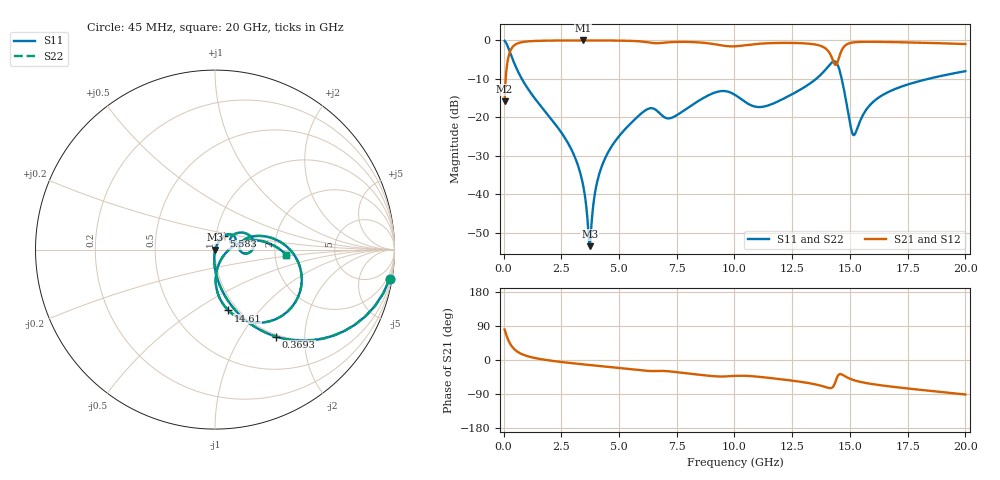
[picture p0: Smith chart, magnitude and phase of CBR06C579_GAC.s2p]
! S-parameter model data by Modelithics Inc.  support@modelithics.com 813-866-6335  Tampa FL USA
! S-Parameter data specifications:
! Substrate: 20-mil Rogers 4350B, substrate thickness, H=0.508mm, Dielectric constant, Er=3.75
! PCB Mounting Pad Footprint: Pad width, PadW=0.85mm , Pad length, PadL=0.64mm , Pad gap, PadG (edge-to-edge)=0.62mm , Reference planes=1.9mm apart
#  GHz  S  MA  R 50
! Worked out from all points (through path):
!   801 points, 45 MHz to 20 GHz, reference 50 ohm
!   highest |S21| = -0.02 dB at 3.437 GHz (marker M1); lowest = -15.8 dB at 45 MHz (marker M2)
!   group delay of S21, straight-line fit = 13.8 ps
!   lowest |S11| = -53.5 dB at 3.737 GHz (marker M3), VSWR 1.00, Z = 50.2 - j0.0167 ohm
!   |S11| at or under -10 dB: 790.3 MHz to 13.54 GHz (12.75 GHz wide, 178 % of centre); 14.64 GHz to 18.4 GHz (3.756 GHz wide, 22.7 % of centre)
!   |S22| runs from -53.5 to -0.1 dB; largest |S21 - S12| = 0
!   S11 on the Smith chart (normalised r, x): 45 MHz: 1, -12; 369.3 MHz: 0.97, -1.45; 5.583 GHz: 1.09, +0.16; 14.61 GHz: 0.91, -0.70; 20 GHz: 2.31, -0.15
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0.045  0.9868 -9.5  0.1616 80.5  0.1616 80.5  0.9868 -9.5
0.194662  0.8151 -36.1  0.5788 53.9  0.5788 53.9  0.8151 -36.1
0.369269  0.5933 -54.9  0.8043 35.1  0.8043 35.1  0.5933 -54.9
1.067694  0.2316 -80.1  0.9717 9.6  0.9717 9.6  0.2316 -80.1
2.738925  0.04897 -95.1  0.9971 -6.9  0.9971 -6.9  0.04897 -95.1
3.387462  0.01571 -94.4  0.9979 -11.1  0.9979 -11.1  0.01571 -94.4
3.43735  0.0134 -93.4  0.9979 -11.4  0.9979 -11.4  0.0134 -93.4
3.736675  0.002102 -4.6  0.9977 -13.3  0.9977 -13.3  0.002102 -4.6
4.011056  0.01258 64.3  0.9974 -14.9  0.9974 -14.9  0.01258 64.3
4.285437  0.02442 66.9  0.9967 -16.6  0.9967 -16.6  0.02442 66.9
5.582512  0.08774 57.3  0.9837 -24.7  0.9837 -24.7  0.08774 57.3
6.704981  0.1169 20.5  0.9194 -28.7  0.9194 -28.7  0.1169 20.5
10.0225  0.1954 -4.3  0.8376 -41.9  0.8376 -41.9  0.1954 -4.3
11.24474  0.1372 7.9  0.9115 -45.5  0.9115 -45.5  0.1372 7.9
13.36496  0.2879 14.8  0.8964 -62.6  0.8964 -62.6  0.2879 14.8
14.21305  0.515 -20.3  0.6012 -73.4  0.6012 -73.4  0.515 -20.3
14.43754  0.5018 -52.9  0.499 -46.7  0.499 -46.7  0.5018 -52.9
14.61215  0.347 -77.6  0.7088 -37.4  0.7088 -37.4  0.347 -77.6
15.16091  0.05861 -37.3  0.9427 -53.1  0.9427 -53.1  0.05861 -37.3
15.83439  0.1405 15.0  0.9588 -62.2  0.9588 -62.2  0.1405 15.0
16.68248  0.2145 14.1  0.9518 -69.4  0.9518 -69.4  0.2145 14.1
20  0.3977 -3.9  0.8966 -91.1  0.8966 -91.1  0.3977 -3.9
